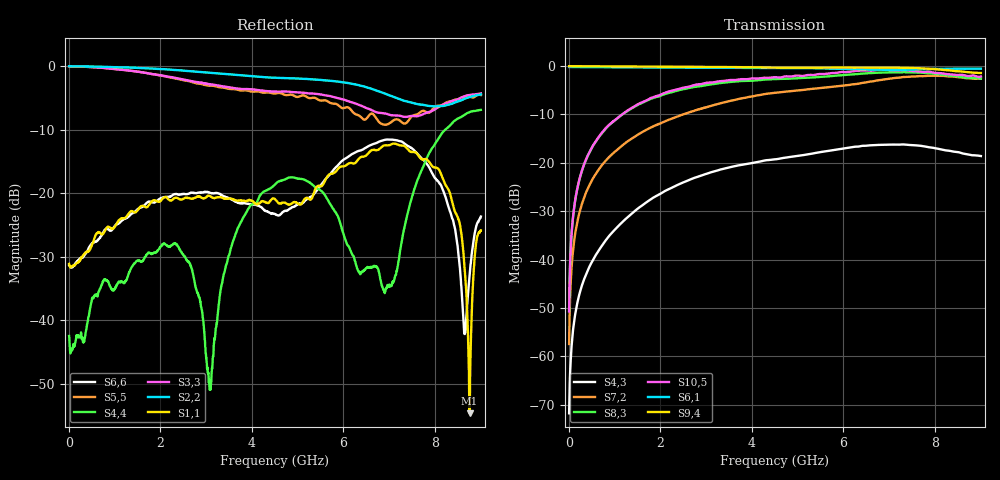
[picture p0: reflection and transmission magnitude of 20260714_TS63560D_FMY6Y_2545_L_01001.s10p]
# GHz S DB R 50
! CMT, SN0916, 25263762, 26.7.0
! Date: 15.07.2026 13:37:55
! Data: Format
! Freq S1.1:dB/Ang S1.2:dB/Ang S1.3:dB/Ang S1.4:dB/Ang S1.5:dB/Ang S1.6:dB/Ang S1.7:dB/Ang S1.8:dB/Ang S1.9:dB/Ang S1.10:dB/Ang
!  S2.1:dB/Ang S2.2:dB/Ang S2.3:dB/Ang S2.4:dB/Ang S2.5:dB/Ang S2.6:dB/Ang S2.7:dB/Ang S2.8:dB/Ang S2.9:dB/Ang S2.10:dB/Ang
!  S3.1:dB/Ang S3.2:dB/Ang S3.3:dB/Ang S3.4:dB/Ang S3.5:dB/Ang S3.6:dB/Ang S3.7:dB/Ang S3.8:dB/Ang S3.9:dB/Ang S3.10:dB/Ang
!  S4.1:dB/Ang S4.2:dB/Ang S4.3:dB/Ang S4.4:dB/Ang S4.5:dB/Ang S4.6:dB/Ang S4.7:dB/Ang S4.8:dB/Ang S4.9:dB/Ang S4.10:dB/Ang
!  S5.1:dB/Ang S5.2:dB/Ang S5.3:dB/Ang S5.4:dB/Ang S5.5:dB/Ang S5.6:dB/Ang S5.7:dB/Ang S5.8:dB/Ang S5.9:dB/Ang S5.10:dB/Ang
!  S6.1:dB/Ang S6.2:dB/Ang S6.3:dB/Ang S6.4:dB/Ang S6.5:dB/Ang S6.6:dB/Ang S6.7:dB/Ang S6.8:dB/Ang S6.9:dB/Ang S6.10:dB/Ang
!  S7.1:dB/Ang S7.2:dB/Ang S7.3:dB/Ang S7.4:dB/Ang S7.5:dB/Ang S7.6:dB/Ang S7.7:dB/Ang S7.8:dB/Ang S7.9:dB/Ang S7.10:dB/Ang
!  S8.1:dB/Ang S8.2:dB/Ang S8.3:dB/Ang S8.4:dB/Ang S8.5:dB/Ang S8.6:dB/Ang S8.7:dB/Ang S8.8:dB/Ang S8.9:dB/Ang S8.10:dB/Ang
!  S9.1:dB/Ang S9.2:dB/Ang S9.3:dB/Ang S9.4:dB/Ang S9.5:dB/Ang S9.6:dB/Ang S9.7:dB/Ang S9.8:dB/Ang S9.9:dB/Ang S9.10:dB/Ang
!  S10.1:dB/Ang S10.2:dB/Ang S10.3:dB/Ang S10.4:dB/Ang S10.5:dB/Ang S10.6:dB/Ang S10.7:dB/Ang S10.8:dB/Ang S10.9:dB/Ang S10.10:dB/Ang
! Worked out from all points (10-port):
!   2001 points, 10 MHz to 9 GHz, reference 50 ohm
!   strongest paths, dB at 10 MHz, 2.257 GHz, 4.505 GHz, 6.753 GHz, 9 GHz:
!     S9,4: -0.1, -0.2, -0.4, -0.4, -1.5
!     S6,1: -0.2, -0.4, -0.5, -0.8, -0.6
!     S10,5: -50.7, -5.1, -2.4, -0.8, -2.2
!     S8,3: -50.7, -5.4, -2.7, -1.4, -2.6
!     S7,2: -57.4, -10.9, -5.6, -3.0, -2.7
!     S4,3: -71.8, -25.2, -19.3, -16.3, -18.6
!   lowest |S11| = -54.7 dB at 8.753 GHz (marker M1), VSWR 1.00, Z = 50 - j0.184 ohm
!   |S11| at or under -10 dB: start of sweep to end of sweep
